(* Logix 5000 AddOnInstructionDefinition export AMCI_MA_Program_Assembed_Move; software revision 20.05 *)

TYPE AMCI_Motion_Axis_Output_Data :
STRUCT
   Control_Word_0 : INT;
   Control_Word_1 : INT;
   Position_or_Distance : DINT;
   Programmed_Speed : DINT;
   Acceleration : INT;
   Deceleration : INT;
   Output_Word_8 : INT;
   Output_Word_9 : INT;
END_STRUCT
END_TYPE

TYPE AMCI_Motion_Axis_Input_Data :
STRUCT
   Moving_CW : BOOL;
   Moving_CCW : BOOL;
   In_Hold_State : BOOL;
   Stopped : BOOL;
   At_Home : BOOL;
   Accelerating : BOOL;
   Decelerating : BOOL;
   Move_Complete : BOOL;
   Status_Word_0_Bit_8 : BOOL;
   Status_Word_0_Bit_9 : BOOL;
   Position_Invalid : BOOL;
   Input_Error : BOOL;
   Command_Error : BOOL;
   Configuration_Error : BOOL;
   Module_OK : BOOL;
   Mode_Flag : BOOL;
   IN1_Active : BOOL;
   IN2_Active : BOOL;
   IN3_Active : BOOL;
   IN4_Active : BOOL;
   Status_Word_1_Bit_4 : BOOL;
   Status_Word_1_Bit_5 : BOOL;
   Connection_Was_Lost : BOOL;
   Driver_Fault : BOOL;
   Status_Word_1_Bit_8 : BOOL;
   Invalid_Jog_Change : BOOL;
   Status_Word_1_Bit_10 : BOOL;
   Heartbeat_Bit : BOOL;
   Status_Word_1_Bit_12 : BOOL;
   Status_Word_1_Bit_13 : BOOL;
   Stall_Detected : BOOL;
   Drive_Is_Enabled : BOOL;
   Motor_Position : DINT;
   Encoder_Position : DINT;
   Trapped_Encoder_Position : DINT;
   Input_Word_8 : INT;
   Input_Word_9 : INT;
END_STRUCT
END_TYPE

ADD_ON_INSTRUCTION AMCI_MA_Program_Assembed_Move   (* revision 1.0, vendor AMCI, ExecuteEnableInFalse *)
// Program Assembled Moves for SD and SMD devices.  Will not work with SV integrated servo devices.
// Help:
// MOTION AXIS PROGRAM ASSEMBLED MOVE
// This AOIs will only work with the SD and SMD motion devices.  The SV motion devices do not support Assembled Moves.
// Up to 16 segments can be programmed into an Assembled Move.
// AXIS INPUT DATA:  Input data from AMCI motion device.   Uses the AMCI_Motion_Axis_Input_Data User Defined Data Type.
// AXIS OUTPUT DATA; Output data from the AOI to the AMCI motion device.   Uses the AMCI_Motion_Axis_Output_Data User Defined Data Type.
// NUMBER_OF_SEGMENTS: Number of Move segments, range of 2 to 16.
// SEGMENT_X_DISTANCE: The relative number of steps to move in the “X” segment.
// SEGMENT_X_PROGRAMMED_SPEED:   The target speed of the “X” segment
// SEGMENT_X_ACCELERATION: If the programmed speed of the previous segment is less than the                                                      programmed speed of the current segment, the acceleration is used as the                                                      rate of change of the speed between the two segments.
// SEGMENT_X_DECELERATION: If the programmed speed of the previous segment is greater than the                                                       programmed speed of the current segment, the deceleration is used as the                                                       rate of change of the speed between the two segments.
// EN (Enable) Set when rung is true, Reset when rung is false
// ER (Error) Set when a command or input error failed to clear.  Reset when the rung is false.
// ASSEMBLED_MOVE_PROGRAMMED: Set when All segments of the Assembled Move have been                                                                 programmed.  Reset when the rung is false.
VAR_IN_OUT
   Axis_Input_data : AMCI_Motion_Axis_Input_Data; {required}
   Axis_Output_data : AMCI_Motion_Axis_Output_Data; {required}
END_VAR
VAR_INPUT
   Number_of_Segments : DINT; {required}
   Segment_1_Distance : DINT; {required}
   Segment_1_Programmed_Speed : DINT; {required}
   Segment_1_Acceleration : INT; {required}
   Segment_1_Deceleration : INT; {required}
   Segment_2_Distance : DINT; {required}
   Segment_2_Programmed_Speed : DINT; {required}
   Segment_2_Acceleration : INT; {required}
   Segment_2_Deceleration : INT; {required}
   Segment_3_Distance : DINT; {required}
   Segment_3_Programmed_Speed : DINT; {required}
   Segment_3_Acceleration : INT; {required}
   Segment_3_Deceleration : INT; {required}
   Segment_4_Distance : DINT; {required}
   Segment_4_Programmed_Speed : DINT; {required}
   Segment_4_Acceleration : INT; {required}
   Segment_4_Deceleration : INT; {required}
   Segment_5_Distance : DINT; {required}
   Segment_5_Programmed_Speed : DINT; {required}
   Segment_5_Acceleration : INT; {required}
   Segment_5_Deceleration : INT; {required}
   Segment_6_Distance : DINT; {required}
   Segment_6_Programmed_Speed : DINT; {required}
   Segment_6_Acceleration : INT; {required}
   Segment_6_Deceleration : INT; {required}
   Segment_7_Distance : DINT; {required}
   Segment_7_Programmed_Speed : DINT; {required}
   Segment_7_Acceleration : INT; {required}
   Segment_7_Deceleration : INT; {required}
   Segment_8_Distance : DINT; {required}
   Segment_8_Programmed_Speed : DINT; {required}
   Segment_8_Acceleration : INT; {required}
   Segment_8_Deceleration : INT; {required}
   Segment_9_Distance : DINT; {required}
   Segment_9_Programmed_Speed : DINT; {required}
   Segment_9_Acceleration : INT; {required}
   Segment_9_Deceleration : INT; {required}
   Segment_10_Distance : DINT; {required}
   Segment_10_Programmed_Speed : DINT; {required}
   Segment_10_Acceleration : INT; {required}
   Segment_10_Deceleration : INT; {required}
   Segment_11_Distance : DINT; {required}
   Segment_11_Programmed_Speed : DINT; {required}
   Segment_11_Acceleration : INT; {required}
   Segment_11_Deceleration : INT; {required}
   Segment_12_Distance : DINT; {required}
   Segment_12_Programmed_Speed : DINT; {required}
   Segment_12_Acceleration : INT; {required}
   Segment_12_Deceleration : INT; {required}
   Segment_13_Distance : DINT; {required}
   Segment_13_Programmed_Speed : DINT; {required}
   Segment_13_Acceleration : INT; {required}
   Segment_13_Deceleration : INT; {required}
   Segment_14_Distance : DINT; {required}
   Segment_14_Programmed_Speed : DINT; {required}
   Segment_14_Acceleration : INT; {required}
   Segment_14_Deceleration : INT; {required}
   Segment_15_Distance : DINT; {required}
   Segment_15_Programmed_Speed : DINT; {required}
   Segment_15_Acceleration : INT; {required}
   Segment_15_Deceleration : INT; {required}
   Segment_16_Distance : DINT; {required}
   Segment_16_Programmed_Speed : DINT; {required}
   Segment_16_Acceleration : INT; {required}
   Segment_16_Deceleration : INT; {required}
END_VAR
VAR_OUTPUT
   EN : BOOL; {access Read Only, visible}
   ER : BOOL; {access Read Only, visible}
   Assembled_Move_Programmed : BOOL; {access Read Only, visible}
END_VAR
VAR
   command_data_block : INT[10];
        [0]   // Command Bits MSW
        [1]   // Command Bits LSW
        [2]   // Upper Target Position
        [3]   // Lower Target Position
        [4]   // Upper Programmed Speed
        [5]   // Lower Programmed Speed
   Assembled_Move_setup : INT[10] := ([0] := 2048, [1] := -32768); {access None}
   Assembled_Move_counter : COUNTER := (PRE := 5); {access None}
        .ACC   // Controls which segment is sent to the Motion Axis Device
   comment_coil : BOOL; {access None}
END_VAR

ROUTINE EnableInFalse   (* ladder *)
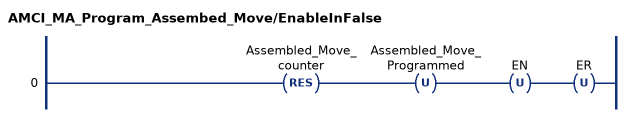
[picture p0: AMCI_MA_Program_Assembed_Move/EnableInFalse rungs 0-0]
   0: RES(Assembled_Move_counter)OTU(Assembled_Move_Programmed)OTU(EN)OTU(ER);
END_ROUTINE

ROUTINE Logic   (* ladder *)
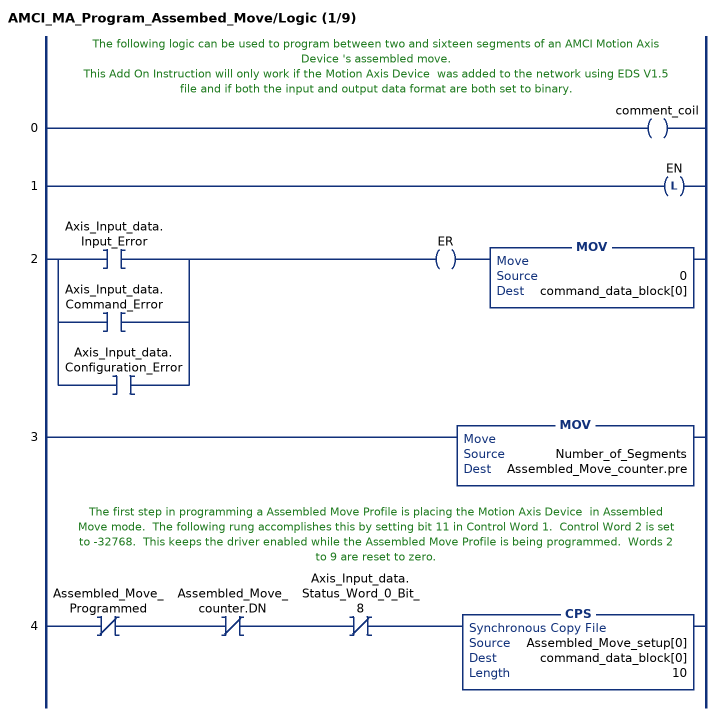
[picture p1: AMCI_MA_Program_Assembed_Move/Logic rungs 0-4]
   // The following logic can be used to program between two and sixteen segments of an AMCI Motion Axis Device 's assembled move.
   // This Add On Instruction will only work if the Motion Axis Device  was added to the network using EDS V1.5 file and if both the input and output data format are both set to binary.
   0: OTE(comment_coil);
   1: OTL(EN);
   2: [XIC(Axis_Input_data.Input_Error) ,XIC(Axis_Input_data.Command_Error) ,XIC(Axis_Input_data.Configuration_Error) ]OTE(ER)MOV(0,command_data_block[0]);
   3: MOV(Number_of_Segments,Assembled_Move_counter.pre);
   // The first step in programming a Assembled Move Profile is placing the Motion Axis Device  in Assembled Move mode.  The following rung accomplishes this by setting bit 11 in Control Word 1.  Control Word 2 is set to -32768.  This keeps the driver enabled while the Assembled Move Profile is being programmed.  Words 2 to 9 are reset to zero.
   4: XIO(Assembled_Move_Programmed)XIO(Assembled_Move_counter.DN)XIO(Axis_Input_data.Status_Word_0_Bit_8)CPS(Assembled_Move_setup[0],command_data_block[0],10);
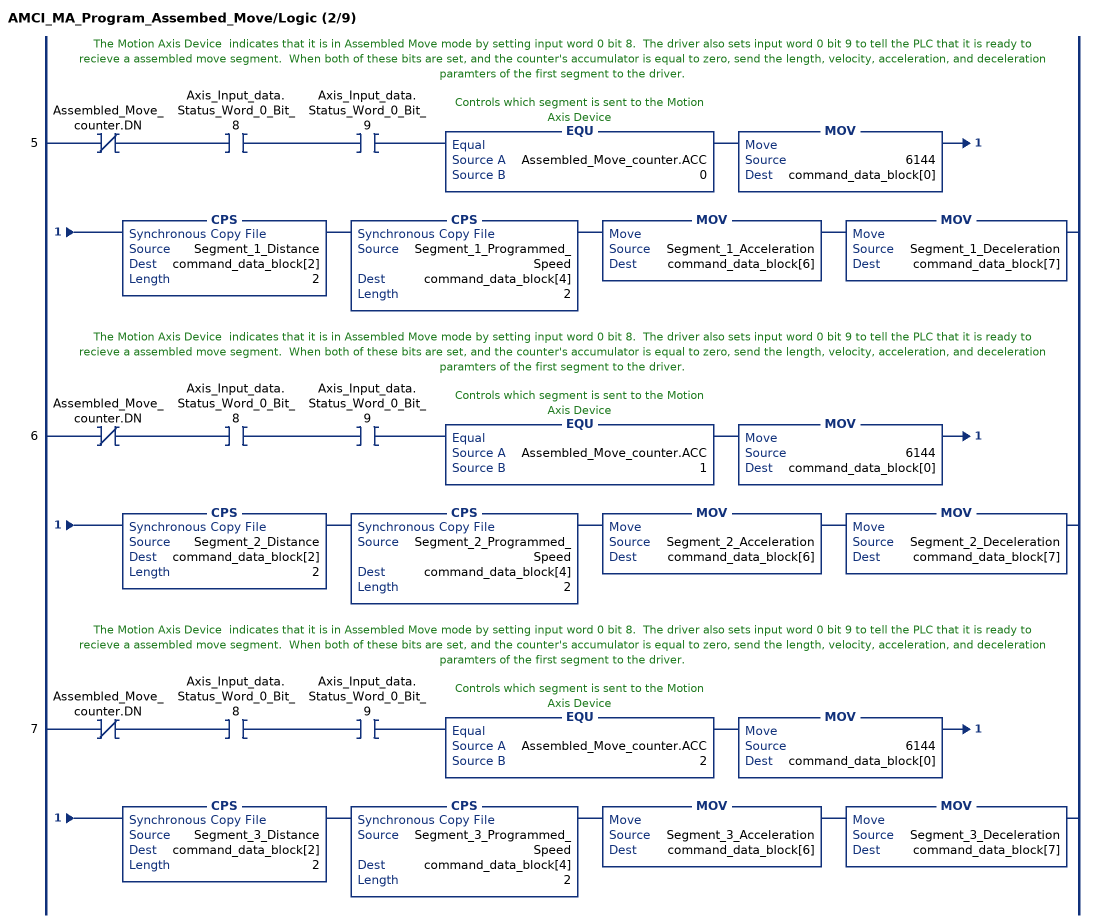
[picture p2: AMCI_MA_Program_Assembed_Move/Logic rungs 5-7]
   // The Motion Axis Device  indicates that it is in Assembled Move mode by setting input word 0 bit 8.  The driver also sets input word 0 bit 9 to tell the PLC that it is ready to recieve a assembled move segment.  When both of these bits are set, and the counter's accumulator is equal to zero, send the length, velocity, acceleration, and deceleration paramters of the first segment to the driver.
   5: XIO(Assembled_Move_counter.DN)XIC(Axis_Input_data.Status_Word_0_Bit_8)XIC(Axis_Input_data.Status_Word_0_Bit_9)EQU(Assembled_Move_counter.ACC,0)MOV(6144,command_data_block[0])CPS(Segment_1_Distance,command_data_block[2],2)CPS(Segment_1_Programmed_Speed,command_data_block[4],2)MOV(Segment_1_Acceleration,command_data_block[6])MOV(Segment_1_Deceleration,command_data_block[7]);
   // The Motion Axis Device  indicates that it is in Assembled Move mode by setting input word 0 bit 8.  The driver also sets input word 0 bit 9 to tell the PLC that it is ready to recieve a assembled move segment.  When both of these bits are set, and the counter's accumulator is equal to zero, send the length, velocity, acceleration, and deceleration paramters of the first segment to the driver.
   6: XIO(Assembled_Move_counter.DN)XIC(Axis_Input_data.Status_Word_0_Bit_8)XIC(Axis_Input_data.Status_Word_0_Bit_9)EQU(Assembled_Move_counter.ACC,1)MOV(6144,command_data_block[0])CPS(Segment_2_Distance,command_data_block[2],2)CPS(Segment_2_Programmed_Speed,command_data_block[4],2)MOV(Segment_2_Acceleration,command_data_block[6])MOV(Segment_2_Deceleration,command_data_block[7]);
   // The Motion Axis Device  indicates that it is in Assembled Move mode by setting input word 0 bit 8.  The driver also sets input word 0 bit 9 to tell the PLC that it is ready to recieve a assembled move segment.  When both of these bits are set, and the counter's accumulator is equal to zero, send the length, velocity, acceleration, and deceleration paramters of the first segment to the driver.
   7: XIO(Assembled_Move_counter.DN)XIC(Axis_Input_data.Status_Word_0_Bit_8)XIC(Axis_Input_data.Status_Word_0_Bit_9)EQU(Assembled_Move_counter.ACC,2)MOV(6144,command_data_block[0])CPS(Segment_3_Distance,command_data_block[2],2)CPS(Segment_3_Programmed_Speed,command_data_block[4],2)MOV(Segment_3_Acceleration,command_data_block[6])MOV(Segment_3_Deceleration,command_data_block[7]);
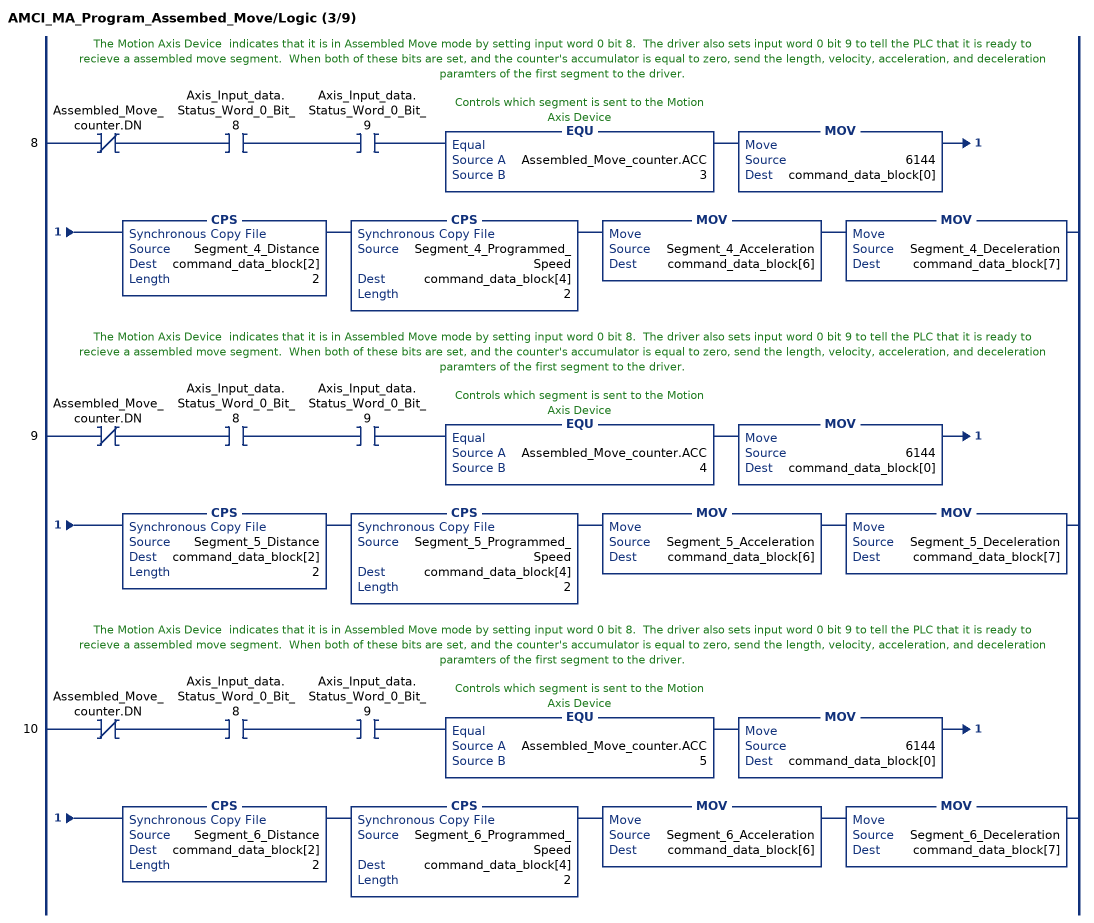
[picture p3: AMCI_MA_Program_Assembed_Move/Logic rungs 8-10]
   // The Motion Axis Device  indicates that it is in Assembled Move mode by setting input word 0 bit 8.  The driver also sets input word 0 bit 9 to tell the PLC that it is ready to recieve a assembled move segment.  When both of these bits are set, and the counter's accumulator is equal to zero, send the length, velocity, acceleration, and deceleration paramters of the first segment to the driver.
   8: XIO(Assembled_Move_counter.DN)XIC(Axis_Input_data.Status_Word_0_Bit_8)XIC(Axis_Input_data.Status_Word_0_Bit_9)EQU(Assembled_Move_counter.ACC,3)MOV(6144,command_data_block[0])CPS(Segment_4_Distance,command_data_block[2],2)CPS(Segment_4_Programmed_Speed,command_data_block[4],2)MOV(Segment_4_Acceleration,command_data_block[6])MOV(Segment_4_Deceleration,command_data_block[7]);
   // The Motion Axis Device  indicates that it is in Assembled Move mode by setting input word 0 bit 8.  The driver also sets input word 0 bit 9 to tell the PLC that it is ready to recieve a assembled move segment.  When both of these bits are set, and the counter's accumulator is equal to zero, send the length, velocity, acceleration, and deceleration paramters of the first segment to the driver.
   9: XIO(Assembled_Move_counter.DN)XIC(Axis_Input_data.Status_Word_0_Bit_8)XIC(Axis_Input_data.Status_Word_0_Bit_9)EQU(Assembled_Move_counter.ACC,4)MOV(6144,command_data_block[0])CPS(Segment_5_Distance,command_data_block[2],2)CPS(Segment_5_Programmed_Speed,command_data_block[4],2)MOV(Segment_5_Acceleration,command_data_block[6])MOV(Segment_5_Deceleration,command_data_block[7]);
   // The Motion Axis Device  indicates that it is in Assembled Move mode by setting input word 0 bit 8.  The driver also sets input word 0 bit 9 to tell the PLC that it is ready to recieve a assembled move segment.  When both of these bits are set, and the counter's accumulator is equal to zero, send the length, velocity, acceleration, and deceleration paramters of the first segment to the driver.
   10: XIO(Assembled_Move_counter.DN)XIC(Axis_Input_data.Status_Word_0_Bit_8)XIC(Axis_Input_data.Status_Word_0_Bit_9)EQU(Assembled_Move_counter.ACC,5)MOV(6144,command_data_block[0])CPS(Segment_6_Distance,command_data_block[2],2)CPS(Segment_6_Programmed_Speed,command_data_block[4],2)MOV(Segment_6_Acceleration,command_data_block[6])MOV(Segment_6_Deceleration,command_data_block[7]);
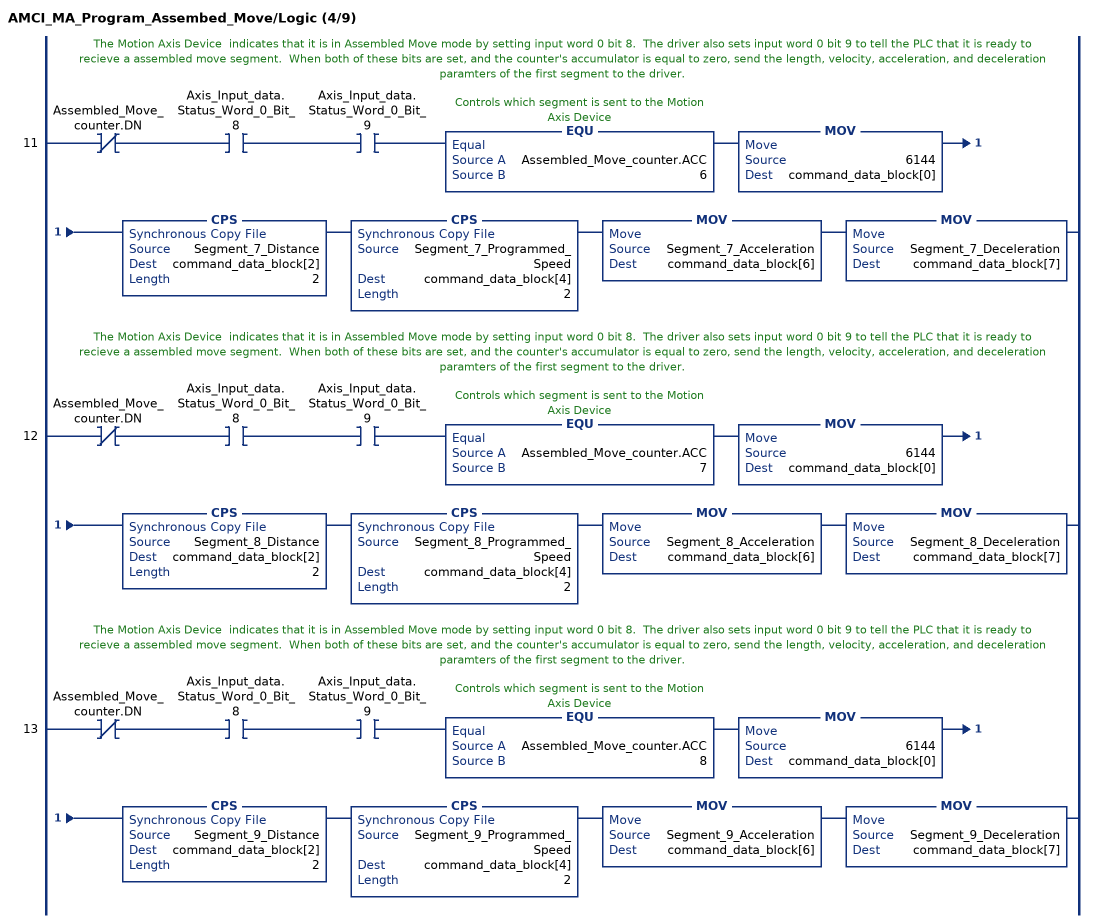
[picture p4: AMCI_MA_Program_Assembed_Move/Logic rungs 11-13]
   // The Motion Axis Device  indicates that it is in Assembled Move mode by setting input word 0 bit 8.  The driver also sets input word 0 bit 9 to tell the PLC that it is ready to recieve a assembled move segment.  When both of these bits are set, and the counter's accumulator is equal to zero, send the length, velocity, acceleration, and deceleration paramters of the first segment to the driver.
   11: XIO(Assembled_Move_counter.DN)XIC(Axis_Input_data.Status_Word_0_Bit_8)XIC(Axis_Input_data.Status_Word_0_Bit_9)EQU(Assembled_Move_counter.ACC,6)MOV(6144,command_data_block[0])CPS(Segment_7_Distance,command_data_block[2],2)CPS(Segment_7_Programmed_Speed,command_data_block[4],2)MOV(Segment_7_Acceleration,command_data_block[6])MOV(Segment_7_Deceleration,command_data_block[7]);
   // The Motion Axis Device  indicates that it is in Assembled Move mode by setting input word 0 bit 8.  The driver also sets input word 0 bit 9 to tell the PLC that it is ready to recieve a assembled move segment.  When both of these bits are set, and the counter's accumulator is equal to zero, send the length, velocity, acceleration, and deceleration paramters of the first segment to the driver.
   12: XIO(Assembled_Move_counter.DN)XIC(Axis_Input_data.Status_Word_0_Bit_8)XIC(Axis_Input_data.Status_Word_0_Bit_9)EQU(Assembled_Move_counter.ACC,7)MOV(6144,command_data_block[0])CPS(Segment_8_Distance,command_data_block[2],2)CPS(Segment_8_Programmed_Speed,command_data_block[4],2)MOV(Segment_8_Acceleration,command_data_block[6])MOV(Segment_8_Deceleration,command_data_block[7]);
   // The Motion Axis Device  indicates that it is in Assembled Move mode by setting input word 0 bit 8.  The driver also sets input word 0 bit 9 to tell the PLC that it is ready to recieve a assembled move segment.  When both of these bits are set, and the counter's accumulator is equal to zero, send the length, velocity, acceleration, and deceleration paramters of the first segment to the driver.
   13: XIO(Assembled_Move_counter.DN)XIC(Axis_Input_data.Status_Word_0_Bit_8)XIC(Axis_Input_data.Status_Word_0_Bit_9)EQU(Assembled_Move_counter.ACC,8)MOV(6144,command_data_block[0])CPS(Segment_9_Distance,command_data_block[2],2)CPS(Segment_9_Programmed_Speed,command_data_block[4],2)MOV(Segment_9_Acceleration,command_data_block[6])MOV(Segment_9_Deceleration,command_data_block[7]);
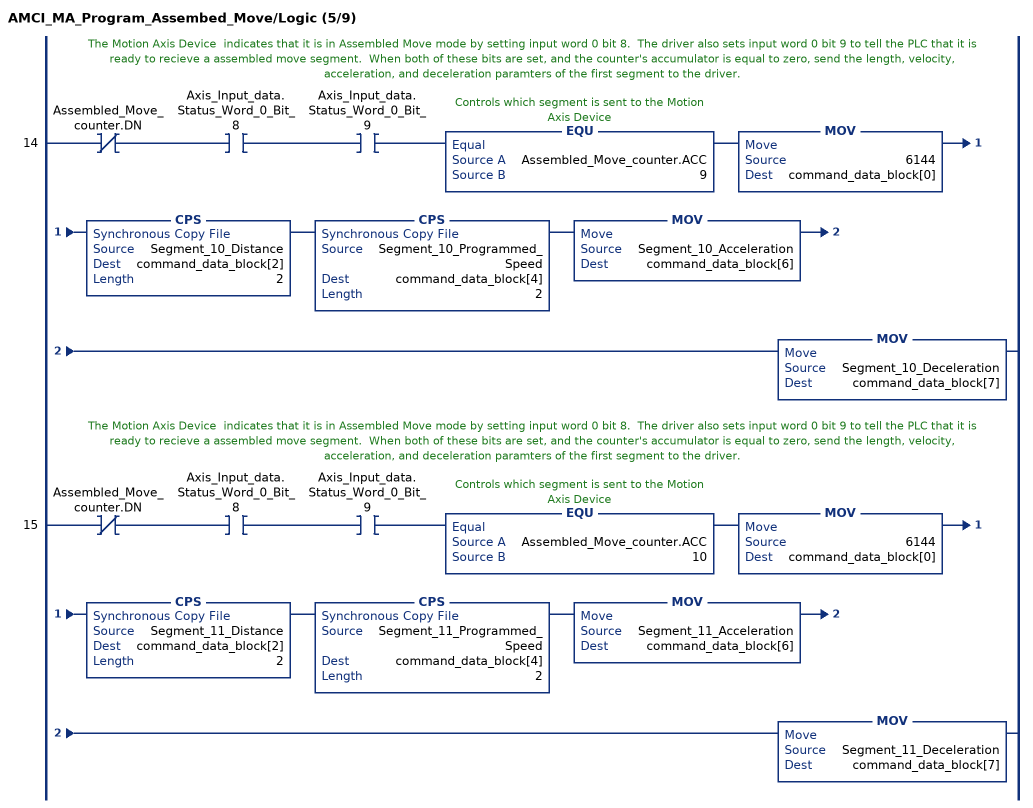
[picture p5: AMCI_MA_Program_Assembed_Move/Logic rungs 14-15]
   // The Motion Axis Device  indicates that it is in Assembled Move mode by setting input word 0 bit 8.  The driver also sets input word 0 bit 9 to tell the PLC that it is ready to recieve a assembled move segment.  When both of these bits are set, and the counter's accumulator is equal to zero, send the length, velocity, acceleration, and deceleration paramters of the first segment to the driver.
   14: XIO(Assembled_Move_counter.DN)XIC(Axis_Input_data.Status_Word_0_Bit_8)XIC(Axis_Input_data.Status_Word_0_Bit_9)EQU(Assembled_Move_counter.ACC,9)MOV(6144,command_data_block[0])CPS(Segment_10_Distance,command_data_block[2],2)CPS(Segment_10_Programmed_Speed,command_data_block[4],2)MOV(Segment_10_Acceleration,command_data_block[6])MOV(Segment_10_Deceleration,command_data_block[7]);
   // The Motion Axis Device  indicates that it is in Assembled Move mode by setting input word 0 bit 8.  The driver also sets input word 0 bit 9 to tell the PLC that it is ready to recieve a assembled move segment.  When both of these bits are set, and the counter's accumulator is equal to zero, send the length, velocity, acceleration, and deceleration paramters of the first segment to the driver.
   15: XIO(Assembled_Move_counter.DN)XIC(Axis_Input_data.Status_Word_0_Bit_8)XIC(Axis_Input_data.Status_Word_0_Bit_9)EQU(Assembled_Move_counter.ACC,10)MOV(6144,command_data_block[0])CPS(Segment_11_Distance,command_data_block[2],2)CPS(Segment_11_Programmed_Speed,command_data_block[4],2)MOV(Segment_11_Acceleration,command_data_block[6])MOV(Segment_11_Deceleration,command_data_block[7]);
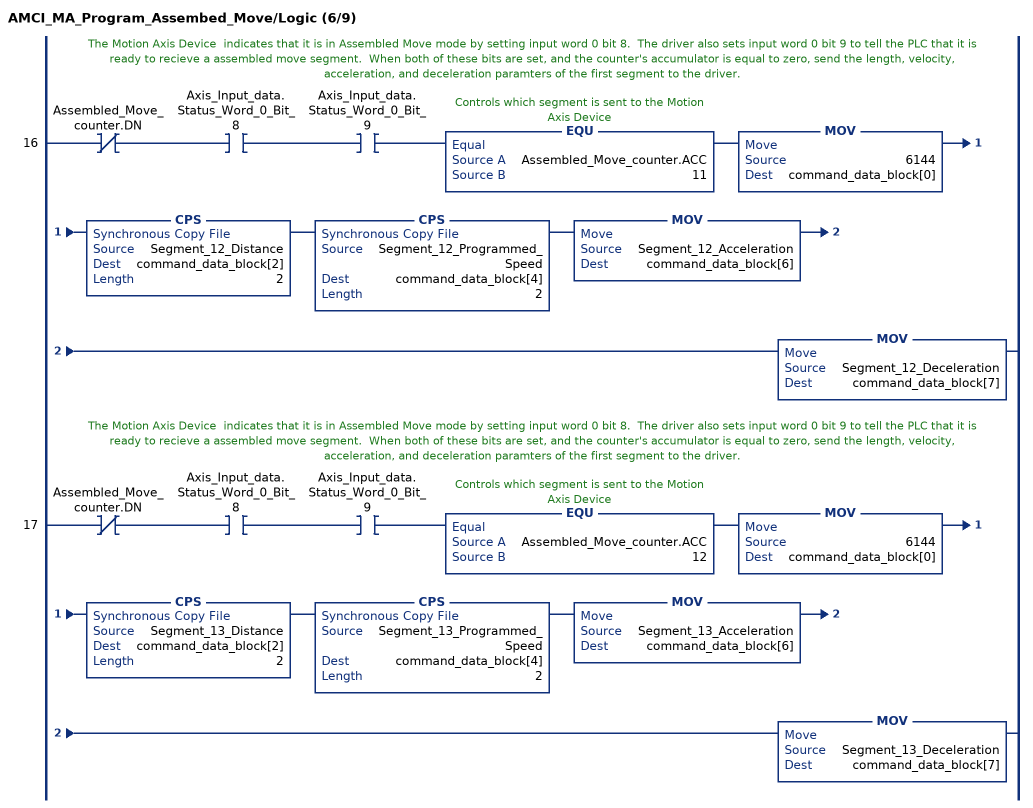
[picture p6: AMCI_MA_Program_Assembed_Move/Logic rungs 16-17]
   // The Motion Axis Device  indicates that it is in Assembled Move mode by setting input word 0 bit 8.  The driver also sets input word 0 bit 9 to tell the PLC that it is ready to recieve a assembled move segment.  When both of these bits are set, and the counter's accumulator is equal to zero, send the length, velocity, acceleration, and deceleration paramters of the first segment to the driver.
   16: XIO(Assembled_Move_counter.DN)XIC(Axis_Input_data.Status_Word_0_Bit_8)XIC(Axis_Input_data.Status_Word_0_Bit_9)EQU(Assembled_Move_counter.ACC,11)MOV(6144,command_data_block[0])CPS(Segment_12_Distance,command_data_block[2],2)CPS(Segment_12_Programmed_Speed,command_data_block[4],2)MOV(Segment_12_Acceleration,command_data_block[6])MOV(Segment_12_Deceleration,command_data_block[7]);
   // The Motion Axis Device  indicates that it is in Assembled Move mode by setting input word 0 bit 8.  The driver also sets input word 0 bit 9 to tell the PLC that it is ready to recieve a assembled move segment.  When both of these bits are set, and the counter's accumulator is equal to zero, send the length, velocity, acceleration, and deceleration paramters of the first segment to the driver.
   17: XIO(Assembled_Move_counter.DN)XIC(Axis_Input_data.Status_Word_0_Bit_8)XIC(Axis_Input_data.Status_Word_0_Bit_9)EQU(Assembled_Move_counter.ACC,12)MOV(6144,command_data_block[0])CPS(Segment_13_Distance,command_data_block[2],2)CPS(Segment_13_Programmed_Speed,command_data_block[4],2)MOV(Segment_13_Acceleration,command_data_block[6])MOV(Segment_13_Deceleration,command_data_block[7]);
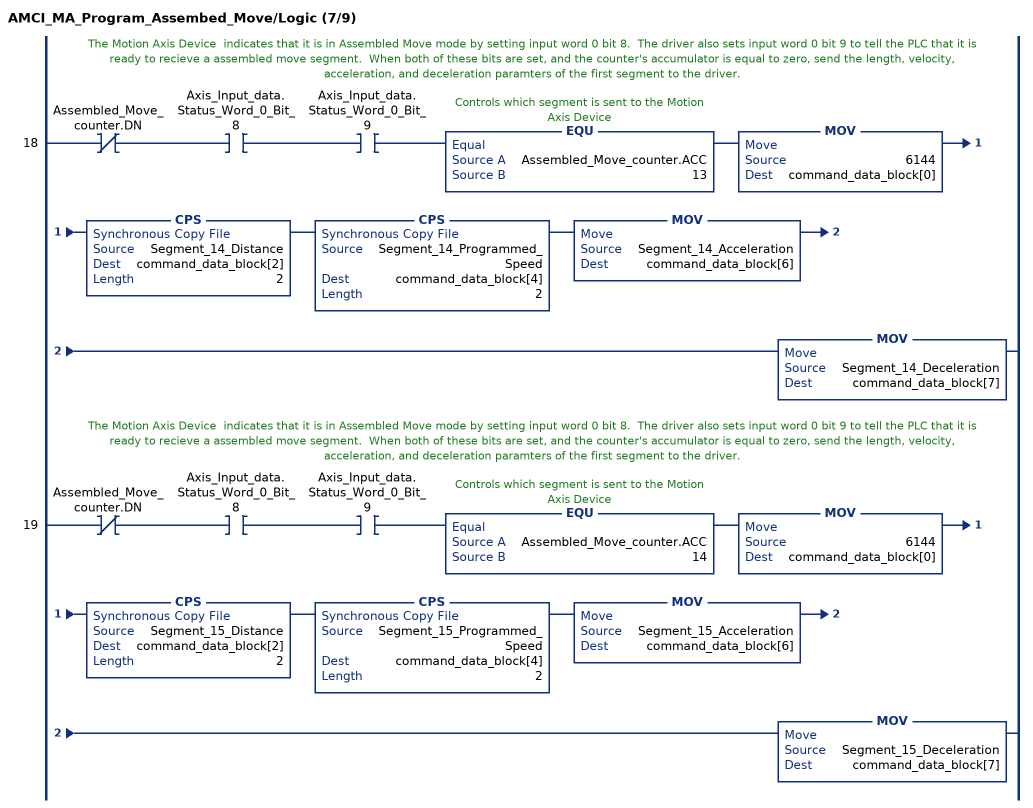
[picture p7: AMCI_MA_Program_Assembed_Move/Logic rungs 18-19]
   // The Motion Axis Device  indicates that it is in Assembled Move mode by setting input word 0 bit 8.  The driver also sets input word 0 bit 9 to tell the PLC that it is ready to recieve a assembled move segment.  When both of these bits are set, and the counter's accumulator is equal to zero, send the length, velocity, acceleration, and deceleration paramters of the first segment to the driver.
   18: XIO(Assembled_Move_counter.DN)XIC(Axis_Input_data.Status_Word_0_Bit_8)XIC(Axis_Input_data.Status_Word_0_Bit_9)EQU(Assembled_Move_counter.ACC,13)MOV(6144,command_data_block[0])CPS(Segment_14_Distance,command_data_block[2],2)CPS(Segment_14_Programmed_Speed,command_data_block[4],2)MOV(Segment_14_Acceleration,command_data_block[6])MOV(Segment_14_Deceleration,command_data_block[7]);
   // The Motion Axis Device  indicates that it is in Assembled Move mode by setting input word 0 bit 8.  The driver also sets input word 0 bit 9 to tell the PLC that it is ready to recieve a assembled move segment.  When both of these bits are set, and the counter's accumulator is equal to zero, send the length, velocity, acceleration, and deceleration paramters of the first segment to the driver.
   19: XIO(Assembled_Move_counter.DN)XIC(Axis_Input_data.Status_Word_0_Bit_8)XIC(Axis_Input_data.Status_Word_0_Bit_9)EQU(Assembled_Move_counter.ACC,14)MOV(6144,command_data_block[0])CPS(Segment_15_Distance,command_data_block[2],2)CPS(Segment_15_Programmed_Speed,command_data_block[4],2)MOV(Segment_15_Acceleration,command_data_block[6])MOV(Segment_15_Deceleration,command_data_block[7]);
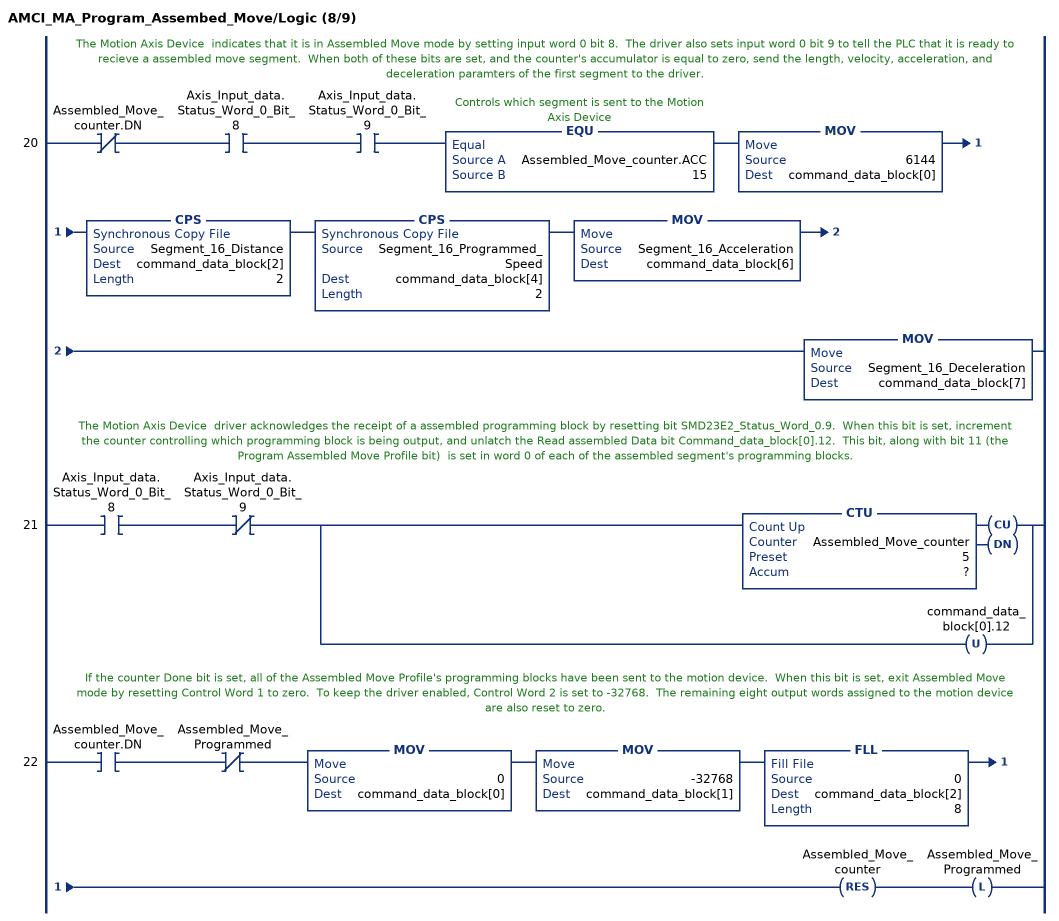
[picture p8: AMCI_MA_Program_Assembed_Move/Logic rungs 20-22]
   // The Motion Axis Device  indicates that it is in Assembled Move mode by setting input word 0 bit 8.  The driver also sets input word 0 bit 9 to tell the PLC that it is ready to recieve a assembled move segment.  When both of these bits are set, and the counter's accumulator is equal to zero, send the length, velocity, acceleration, and deceleration paramters of the first segment to the driver.
   20: XIO(Assembled_Move_counter.DN)XIC(Axis_Input_data.Status_Word_0_Bit_8)XIC(Axis_Input_data.Status_Word_0_Bit_9)EQU(Assembled_Move_counter.ACC,15)MOV(6144,command_data_block[0])CPS(Segment_16_Distance,command_data_block[2],2)CPS(Segment_16_Programmed_Speed,command_data_block[4],2)MOV(Segment_16_Acceleration,command_data_block[6])MOV(Segment_16_Deceleration,command_data_block[7]);
   // The Motion Axis Device  driver acknowledges the receipt of a assembled programming block by resetting bit SMD23E2_Status_Word_0.9.  When this bit is set, increment the counter controlling which programming block is being output, and unlatch the Read assembled Data bit Command_data_block[0].12.  This bit, along with bit 11 (the Program Assembled Move Profile bit)  is set in word 0 of each of the assembled segment's programming blocks.
   21: XIC(Axis_Input_data.Status_Word_0_Bit_8)XIO(Axis_Input_data.Status_Word_0_Bit_9)[CTU(Assembled_Move_counter,?,?) ,OTU(command_data_block[0].12) ];
   // If the counter Done bit is set, all of the Assembled Move Profile's programming blocks have been sent to the motion device.  When this bit is set, exit Assembled Move mode by resetting Control Word 1 to zero.  To keep the driver enabled, Control Word 2 is set to -32768.  The remaining eight output words assigned to the motion device are also reset to zero.
   22: XIC(Assembled_Move_counter.DN)XIO(Assembled_Move_Programmed)MOV(0,command_data_block[0])MOV(-32768,command_data_block[1])FLL(0,command_data_block[2],8)RES(Assembled_Move_counter)OTL(Assembled_Move_Programmed);
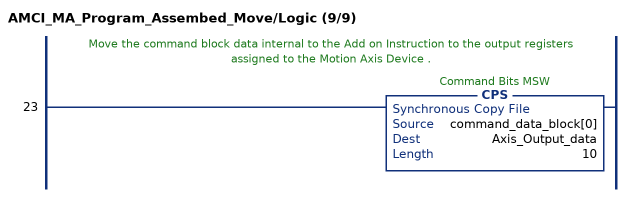
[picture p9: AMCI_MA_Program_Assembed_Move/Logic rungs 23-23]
   // Move the command block data internal to the Add on Instruction to the output registers assigned to the Motion Axis Device .
   23: CPS(command_data_block[0],Axis_Output_data,10);
END_ROUTINE
END_ADD_ON_INSTRUCTION
